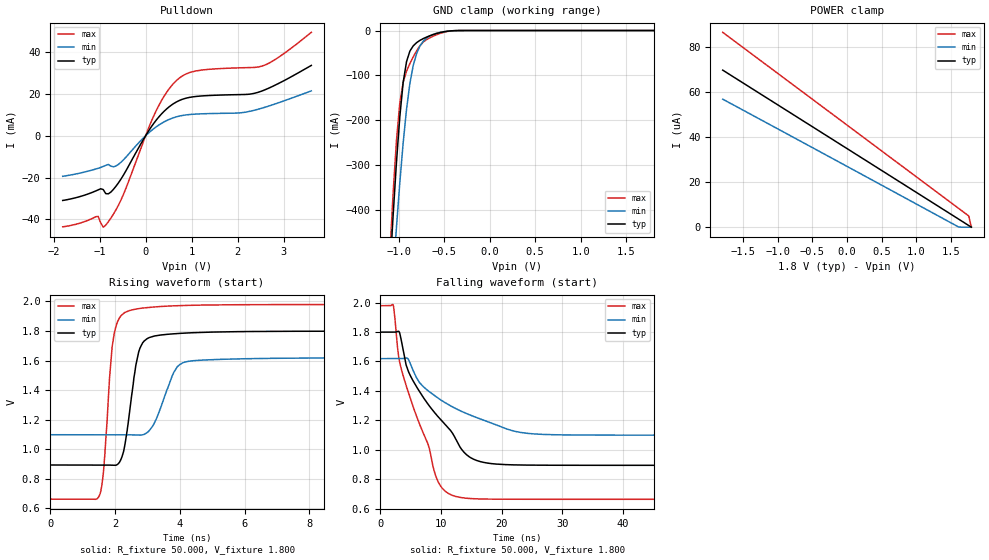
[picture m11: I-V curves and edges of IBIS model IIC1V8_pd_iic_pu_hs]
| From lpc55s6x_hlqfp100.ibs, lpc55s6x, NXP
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|   Model IIC1V8_pd_iic_pu_hs
[Model] IIC1V8_pd_iic_pu_hs
Model_type I/O_open_drain
Polarity   Non-Inverting
Enable   Active-Low
Vinl =  0.540V
Vinh =  1.260V
Vmeas =  0.900V
Cref =  0.0F
Rref =  100.000
Vref =  1.800V
C_comp   2.515pF   2.512pF   2.535pF
C_comp_pulldown   1.736pF   1.670pF   1.792pF
C_comp_power_clamp   0.454pF   0.388pF   0.547pF
[Model Spec]
Vinh   1.260V   1.134V   1.386V
Vinl   0.540V   0.486V   0.594V
Vmeas   0.900V   0.810V   0.990V
Vref   1.800V   1.620V   1.980V
Cref   0.0F   0.0F   0.0F
Rref   100.000   100.000   100.000
[Temperature Range]   25.000   0.125k   -40.000
[Voltage Range]   1.800V   1.620V   1.980V
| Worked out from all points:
|   slope of the pulldown table from 0 to 0.27 V, typ, clamps not added: 31.5 ohm
|   GND clamp passes 1 mA (typ) near -0.44 V on its own axis
|   rising waveform, R_fixture 50.000, V_fixture 1.800: 20-80 % time 350ps typ, 534ps min, 256ps max; typ from 0.894 V to 1.8 V
|   falling waveform, R_fixture 50.000, V_fixture 1.800: 20-80 % time 8.37ns typ, 11.2ns min, 5.71ns max; typ from 1.8 V to 0.894 V
[Pulldown]
|Voltage   I(typ)   I(min)   I(max)
-1.8V     -30.97mA   -19.41mA   -43.61mA
-1.03V    -25.91mA   -15.56mA   -38.59mA
-920mV    -25.75mA   -14.67mA   -43.75mA
-865mV    -27.69mA   -14.16mA   -42.79mA
-700mV    -25.69mA   -14.87mA   -37.58mA
-480mV    -18.8mA    -11.48mA   -28.03mA
235mV     7.619mA    4.356mA    12.23mA
455mV     12.83mA    7.267mA    20.76mA
730mV     16.88mA    9.427mA    27.6mA
1.17V     19mA       10.49mA    31.33mA
2.545V    21.61mA    13.36mA    33.53mA
3.6V      33.71mA    21.52mA    49.57mA
[GND_clamp]
|Voltage   I(typ)   I(min)   I(max)
-1.8V     -3.488A    -3.23A     -3.872A
-1.097V   -545.5mA   -658.5mA   -507mA
-1.06V    -414.6mA   -546.1mA   -365mA
-1.023V   -294.9mA   -439.1mA   -245.9mA
-986mV    -192.4mA   -339.6mA   -162mA
-949mV    -115.6mA   -250.3mA   -115.1mA
-912mV    -69.19mA   -175.2mA   -90.62mA
-838mV    -34.02mA   -77.16mA   -58.5mA
-764mV    -21.82mA   -34.11mA   -33.6mA
-653mV    -11.43mA   -11.65mA   -15.83mA
-431mV    -835.3uA   -879.6uA   -1.141mA
1.8V      0A         0A         0A
[POWER_clamp]
|Voltage   I(typ)   I(min)   I(max)
-1.8V     69.55uA    56.68uA    86.29uA
1.615V    3.579uA    80.87nA    8.337uA
1.763V    715.6nA    0A         4.957uA
1.8V      0A         0A         0A
[Ramp]
| variable   typ   min   max
dV/dt_r   0.543/0.348n   0.312/0.538n   0.790/0.254n
dV/dt_f   0.543/8.372n   0.312/11.242n   0.790/5.707n
R_load = 50.000
[Rising Waveform]
R_fixture= 50.000
V_fixture= 1.800
V_fixture_min= 1.620
V_fixture_max= 1.980
|time   V(typ)   V(min)   V(max)
0s        893.8mV    1.098V     663mV
1.52ns    893.8mV    1.098V     689.6mV
1.65ns    893.9mV    1.098V     863.8mV
1.91ns    892mV      1.098V     1.694V
2.19ns    935.5mV    1.099V     1.905V
2.64ns    1.567V     1.096V     1.948V
2.85ns    1.72V      1.098V     1.955V
3.91ns    1.782V     1.555V     1.971V
5.15ns    1.793V     1.607V     1.976V
600ns     1.799V     1.619V     1.979V
[Falling Waveform]
R_fixture= 50.000
V_fixture= 1.800
V_fixture_min= 1.620
V_fixture_max= 1.980
|time   V(typ)   V(min)   V(max)
0s        1.799V     1.619V     1.979V
2.12ns    1.799V     1.619V     1.984V
2.92ns    1.804V     1.619V     1.664V
3.4ns     1.757V     1.619V     1.558V
4.85ns    1.512V     1.595V     1.362V
6.45ns    1.396V     1.458V     1.177V
9.54ns    1.224V     1.35V      781.9mV
15.39ns   935.4mV    1.226V     667.2mV
30.64ns   894.4mV    1.101V     663.2mV
600ns     893.8mV    1.098V     663mV
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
